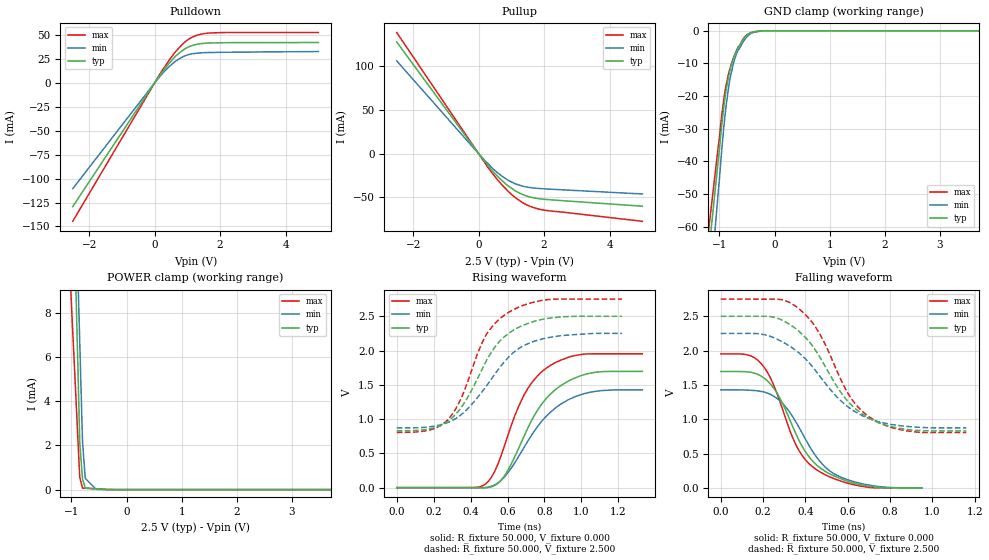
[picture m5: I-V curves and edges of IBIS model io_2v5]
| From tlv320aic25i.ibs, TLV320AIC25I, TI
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[Model]   io_2v5
Model_type I/O
Vinl=7.500E-01
Vinh=1.750E+00
Vref=0.000E+00
Rref=1.000E+06
Cref=2.000E-11
Vmeas=1.250E+00
C_comp   1.070E-12   1.070E-12   1.070E-12
[Voltage Range]   2.500E+00   2.250E+00   2.750E+00
[POWER Clamp Reference]   2.500E+00   2.250E+00   2.750E+00
[GND Clamp Reference]   0.000E+00   0.000E+00   0.000E+00
[Pullup Reference]   2.500E+00   2.250E+00   2.750E+00
[Pulldown Reference]   0.000E+00   0.000E+00   0.000E+00
[Temperature Range]   25   85   -40
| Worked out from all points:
|   slope of the pulldown table from 0 to 0.375 V, typ, clamps not added: 21.4 ohm
|   slope of the pullup table from 0 to 0.375 V, typ, clamps not added: 21.2 ohm
|   GND clamp passes 1 mA (typ) near -0.48 V on its own axis
|   POWER clamp passes 1 mA (typ) near -0.82 V on its own axis
|   rising waveform, R_fixture 50.000, V_fixture 0.000: 20-80 % time 210ps typ, 230ps min, 186ps max; typ from 0 V to 1.7 V
|   falling waveform, R_fixture 50.000, V_fixture 0.000: 20-80 % time 180ps typ, 183ps min, 165ps max; typ from 1.7 V to 0 V
|   rising waveform, R_fixture 50.000, V_fixture 2.500: 20-80 % time 221ps typ, 251ps min, 192ps max; typ from 0.83 V to 2.5 V
|   falling waveform, R_fixture 50.000, V_fixture 2.500: 20-80 % time 225ps typ, 249ps min, 200ps max; typ from 2.5 V to 0.83 V
[GND Clamp]
-2.5V     -282.2mA   -343.8mA   -252mA
-1.02V    -39.29mA   -48.97mA   -35.15mA
-960mV    -29.11mA   -36.7mA    -26.01mA
-900mV    -20.5mA    -26mA      -18.6mA
-840mV    -14.43mA   -18.03mA   -13.54mA
-800mV    -11.46mA   -13.99mA   -11.01mA
-720mV    -7.326mA   -8.411mA   -7.221mA
-660mV    -4.968mA   -5.824mA   -4.891mA
-540mV    -2.01mA    -2.589mA   -1.8mA
-440mV    -589.5uA   -910.3uA   -693.6uA
-220mV    0A         0A         0A
5V        0A         0A         0A
[POWER Clamp]
-2.5V     167.8mA    155.3mA    86.3mA
-1.05V    22.23mA    24.71mA    10.95mA
-850mV    2.14mA     6.693mA    557.3uA
-800mV    484.1uA    2.189mA    65.39uA
-750mV    73.7uA     504.3uA    59.17uA
-550mV    34.39uA    10.79uA    34.25uA
-375mV    0A         0A         12.46uA
5V        0A         0A         0A
[Pullup]
-2.5V     127.7mA    106.1mA    138.5mA
0V        0A         0A         0A
300mV     -14.43mA   -11.94mA   -16.71mA
480mV     -22.14mA   -18.73mA   -25.34mA
700mV     -30.37mA   -25.46mA   -35.19mA
940mV     -38.02mA   -31.21mA   -44.43mA
1.14V     -43.01mA   -34.79mA   -50.86mA
1.5V      -48.88mA   -38.43mA   -59.17mA
1.9V      -51.81mA   -40.02mA   -63.95mA
5V        -60.17mA   -46.18mA   -77.44mA
[Pulldown]
-2.5V     -129.2mA   -110.5mA   -144.6mA
200mV     9.967mA    8.366mA    11.43mA
460mV     21.18mA    17.48mA    24.6mA
640mV     27.95mA    22.74mA    32.71mA
820mV     33.17mA    26.55mA    39.41mA
1V        37.1mA     29.26mA    44.8mA
1.26V     40.22mA    31.06mA    49.57mA
1.68V     41.79mA    31.85mA    52.24mA
5V        42.29mA    32.85mA    52.7mA
[Rising Waveform]
R_fixture = 50.000
V_fixture = 0.000
V_fixture_min = 0.000
V_fixture_max = 0.000
|  time   V(typ)   V(min)   V(max)
0s        0V         0V         0V
470ps     -3.298mV   -900.5uV   33.17mV
520ps     18.46mV    26.82mV    185.1mV
580ps     158.2mV    146.8mV    583.1mV
640ps     456.7mV    365.6mV    1.053V
690ps     752.5mV    588.3mV    1.354V
790ps     1.236V     983.4mV    1.701V
890ps     1.491V     1.221V     1.861V
1.01ns    1.644V     1.367V     1.947V
1.33ns    1.695V     1.427V     1.952V
[Falling Waveform]
R_fixture = 50.000
V_fixture = 0.000
V_fixture_min = 0.000
V_fixture_max = 0.000
|  time   V(typ)   V(min)   V(max)
0s        1.695V     1.427V     1.952V
130ps     1.689V     1.424V     1.935V
200ps     1.611V     1.399V     1.777V
270ps     1.359V     1.293V     1.341V
360ps     754.6mV    933.8mV    598.5mV
400ps     526.7mV    710.7mV    409.6mV
460ps     314.6mV    418.2mV    249.6mV
530ps     180.7mV    215.9mV    140mV
630ps     69.67mV    89.24mV    45.47mV
950ps     0V         0V         0V
[Rising Waveform]
R_fixture = 50.000
V_fixture = 2.500
V_fixture_min = 2.250
V_fixture_max = 2.750
|  time   V(typ)   V(min)   V(max)
0s        829.9mV    873.1mV    805.7mV
180ps     858.4mV    887.7mV    842.4mV
280ps     974.3mV    954.2mV    1V
350ps     1.172V     1.067V     1.31V
480ps     1.825V     1.462V     2.209V
540ps     2.081V     1.689V     2.419V
610ps     2.258V     1.916V     2.564V
700ps     2.385V     2.087V     2.673V
820ps     2.47V      2.188V     2.743V
1.22ns    2.5V       2.25V      2.75V
[Falling Waveform]
R_fixture = 50.000
V_fixture = 2.500
V_fixture_min = 2.250
V_fixture_max = 2.750
|  time   V(typ)   V(min)   V(max)
0s        2.5V       2.25V      2.75V
210ps     2.5V       2.229V     2.749V
290ps     2.444V     2.13V      2.74V
360ps     2.306V     1.99V      2.633V
460ps     1.945V     1.659V     2.283V
560ps     1.424V     1.289V     1.626V
620ps     1.199V     1.138V     1.288V
740ps     957.5mV    968.8mV    962.3mV
910ps     841.2mV    887.5mV    817.9mV
1.16ns    829.9mV    873.1mV    805.7mV
[Ramp]
dV/dt_r   1.018E+00/2.099E-10   8.560E-01/2.298E-10   1.172E+00/1.856E-10
dV/dt_f   1.002E+00/2.247E-10   8.261E-01/2.490E-10   1.167E+00/2.002E-10
R_load = 50
